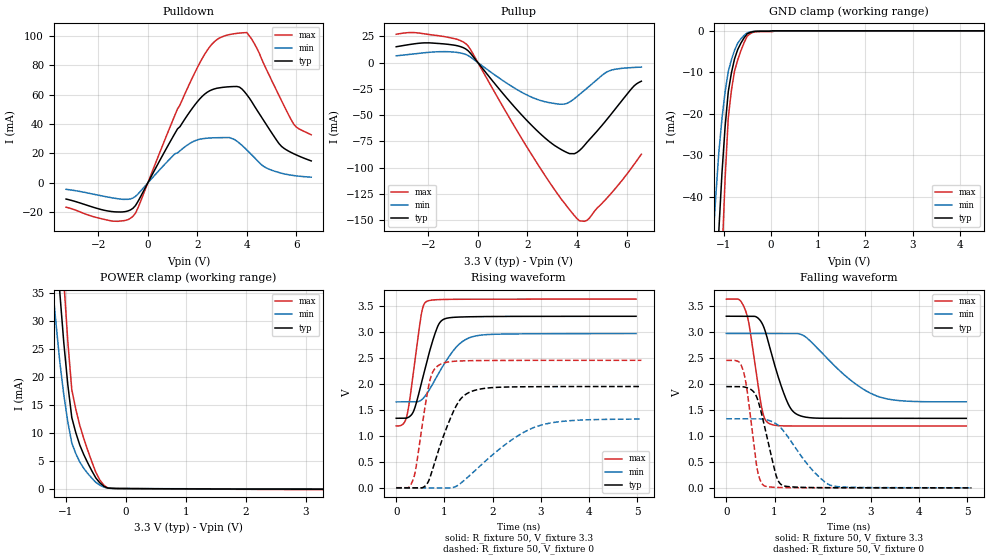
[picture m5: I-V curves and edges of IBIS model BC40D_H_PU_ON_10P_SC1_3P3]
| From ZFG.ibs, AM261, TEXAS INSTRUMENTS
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[Model]   BC40D_H_PU_ON_10P_SC1_3P3
Model_type   I/O
Polarity   Non-Inverting
Enable   Active-Low
Vinl =  0.8V
Vinh =  2V
Cref =  15pF
Rref =  100.0000M
Vref =  0V
Vmeas =  1.65
C_comp   2.157014p   1.997104p   2.250886p
|[Input load] weak_pu_on
|[Output drive] slow
|[supplytol] 10
|[temp] ind
[Model Spec]
Vinl   0.8V   0.8V   0.8V
Vinh   2V   2V   2V
[Temperature Range]   25   125   -40
[Voltage Range]   3.3   2.97   3.63
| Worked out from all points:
|   slope of the pulldown table from 0 to 0.495 V, typ, clamps not added: 31.8 ohm
|   slope of the pullup table from 0 to 0.495 V, typ, clamps not added: 33.8 ohm
|   GND clamp passes 1 mA (typ) near -0.52 V on its own axis
|   POWER clamp passes 1 mA (typ) near -0.43 V on its own axis
|   rising waveform, R_fixture 50, V_fixture 3.3: 20-80 % time 338ps typ, 537ps min, 211ps max; typ from 1.34 V to 3.3 V
|   rising waveform, R_fixture 50, V_fixture 0: 20-80 % time 469ps typ, 1.07ns min, 245ps max; typ from 0 V to 1.95 V
|   falling waveform, R_fixture 50, V_fixture 3.3: 20-80 % time 389ps typ, 938ps min, 235ps max; typ from 3.3 V to 1.34 V
|   falling waveform, R_fixture 50, V_fixture 0: 20-80 % time 295ps typ, 648ps min, 202ps max; typ from 1.95 V to 0.002 V
| Nom Voltages:
|   VDD=1.1001, VDDS=3.3, VDDS18=1.8, ESD_BIASFET=0, VSS=0, VSSS=0
| Min Voltages:
|   VDD=0.99, VDDS=2.97, VDDS18=1.62, ESD_BIASFET=0, VSS=0, VSSS=0
| Max Voltages:
|   VDD=1.21, VDDS=3.63, VDDS18=1.98, ESD_BIASFET=0, VSS=0, VSSS=0
[POWER_clamp]
|   voltage   I(typ)   I(min)   I(max)
-3.3V     446.9mA    419.5mA    603.9mA
-1.233V   56.55mA    37.52mA    80.26mA
-1.167V   45.63mA    29.9mA     65.05mA
-1.1V     35.1mA     22.66mA    50.24mA
-1.033V   26.08mA    16.76mA    37.18mA
-966.7mV  18.62mA    11.92mA    26.33mA
-900mV    12.7mA     8.149mA    17.69mA
-833.3mV  10mA       6.265mA    14.21mA
-766.7mV  7.795mA    4.753mA    11.3mA
-566.7mV  3.199mA    1.871mA    4.823mA
-366.7mV  433.5uA    268.4uA    618.3uA
3.3V      -100.3uA   -83.23uA   -188.3uA
[Pulldown]
|   voltage   I(typ)   I(min)   I(max)
-3.3V     -10.93mA   -4.311mA   -16.48mA
-1.4V     -19.53mA   -10.23mA   -25.96mA
-600mV    -17.23mA   -10.26mA   -22.66mA
1.1V      33.82mA    19.89mA    46.25mA
2V        55.14mA    29.24mA    78.29mA
2.6V      63.35mA    30.61mA    94.45mA
3.2V      65.21mA    30.81mA    100.4mA
3.7V      65.09mA    27.02mA    101.8mA
4V        59.92mA    22.37mA    102.1mA
5.3V      26.68mA    7.058mA    59.31mA
5.9V      19.77mA    5.007mA    39.76mA
6.6V      14.97mA    3.923mA    32.7mA
[Pullup]
|   voltage   I(typ)   I(min)   I(max)
-3.3V     15.12mA    6.498mA    27.02mA
-1.9V     18.73mA    9.943mA    26.53mA
-900mV    16.4mA     9.888mA    22.58mA
-400mV    11.39mA    6.786mA    15.98mA
1.3V      -37.44mA   -21.62mA   -53.74mA
2.4V      -65.08mA   -35.06mA   -96.18mA
3.5V      -84.52mA   -39.53mA   -134mA
4.1V      -83.7mA    -30.35mA   -150.6mA
4.4V      -75.99mA   -24.42mA   -150.3mA
5.3V      -51.41mA   -7.872mA   -126.6mA
6.3V      -22.29mA   -4.606mA   -97.15mA
6.6V      -17.71mA   -4.277mA   -87.2mA
[GND_clamp]
|   voltage   I(typ)   I(min)   I(max)
-3.3V     -787.2mA   -607.8mA   -1.235A
-1.233V   -85.67mA   -52.14mA   -138.8mA
-1.167V   -66.48mA   -40.37mA   -107.8mA
-1.1V     -48.26mA   -29.37mA   -78.02mA
-1.033V   -34.3mA    -21.2mA    -54.63mA
-966.7mV  -23.1mA    -14.67mA   -35.61mA
-900mV    -14.66mA   -9.802mA   -20.96mA
-833.3mV  -10.12mA   -6.954mA   -14.31mA
-700mV    -4.501mA   -2.964mA   -6.982mA
-500mV    -717.7uA   -486.4uA   -1.28mA
100mV     0A         0A         0A
6.6V      0A         0A         0A
[Ramp]
| variable   typ   min   max
dV/dt_f  1.1794646/0.38911142n 0.79416303/0.94543818n  1.4659475/0.2354734n
dV/dt_r  1.1737483/0.47007394n 0.80293565/1.0830673n  1.4758135/0.24585647n
R_load = 50
[Rising Waveform]
R_fixture = 50
V_fixture = 3.3
V_fixture_min = 2.97
V_fixture_max = 3.63
|   time   V(typ)   V(min)   V(max)
0s        1.338V     1.654V     1.191V
223.5ps   1.345V     1.654V     1.394V
362.3ps   1.479V     1.654V     2.258V
520.2ps   2.004V     1.689V     3.334V
633.9ps   2.424V     1.809V     3.586V
816.6ps   3V         2.098V     3.618V
932.2ps   3.208V     2.287V     3.622V
1.275ns   3.284V     2.736V     3.627V
1.573ns   3.291V     2.905V     3.628V
4.974ns   3.3V       2.968V     3.63V
[Rising Waveform]
R_fixture = 50
V_fixture = 0
V_fixture_min = 0
V_fixture_max = 0
|   time   V(typ)   V(min)   V(max)
0s        0V         0V         3.208mV
251.4ps   0V         0V         3.208mV
352.4ps   0V         0V         162.5mV
564.7ps   12.71mV    0V         1.362V
691.5ps   176.1mV    0V         2.042V
908.7ps   811.3mV    0V         2.373V
1.283ns   1.641V     51.72mV    2.439V
1.625ns   1.875V     323.2mV    2.447V
2.957ns   1.947V     1.194V     2.452V
5.084ns   1.949V     1.323V     2.453V
[Falling Waveform]
R_fixture = 50
V_fixture = 3.3
V_fixture_min = 2.97
V_fixture_max = 3.63
|   time   V(typ)   V(min)   V(max)
0s        3.3V       2.969V     3.629V
266.3ps   3.3V       2.969V     3.619V
404.6ps   3.3V       2.969V     3.392V
481.9ps   3.3V       2.969V     3.087V
738ps     3.168V     2.969V     1.521V
886.5ps   2.752V     2.969V     1.239V
1.258ns   1.665V     2.969V     1.192V
1.524ns   1.39V      2.957V     1.191V
3.089ns   1.338V     1.779V     1.19V
4.974ns   1.338V     1.656V     1.19V
[Falling Waveform]
R_fixture = 50
V_fixture = 0
V_fixture_min = 0
V_fixture_max = 0
|   time   V(typ)   V(min)   V(max)
0s        1.948V     1.329V     2.452V
250.2ps   1.948V     1.329V     2.43V
350.9ps   1.944V     1.329V     2.251V
430.5ps   1.927V     1.329V     1.874V
642.3ps   1.717V     1.329V     353mV
785.7ps   1.212V     1.321V     41.5mV
1.033ns   238.9mV    1.234V     10.67mV
1.188ns   41.36mV    1.094V     6.987mV
2.179ns   5.449mV    46.63mV    3.233mV
5.084ns   2.11mV     3.258mV    3.054mV
